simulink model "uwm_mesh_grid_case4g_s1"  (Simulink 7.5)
settings: Solver=ode45  StartTime=0.0  StopTime=8.0  RelTol=1e-4
undefined symbols (not defined in the file or in its folder): D1, Delta, dfilt, DiscIntNeverNeededParam
libraries: powerlib x90, powerlib_extras x24, dsparch4 x6
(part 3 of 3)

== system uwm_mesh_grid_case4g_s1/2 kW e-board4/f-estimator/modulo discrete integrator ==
  In1 : Inport
  Abs : Abs
  Constant1 : Constant  OutDataType=sfix(16)  OutScaling=2^0
  Discrete-Time Integrator : DiscreteIntegrator  ExternalReset=rising  InitialConditionSource=external  SampleTime=dt  OutDataType=fixdt(1, 16)  OutScaling=2^0  UpperSaturationLimit=100  LowerSaturationLimit=-100  ShowStatePort=on  ICPrevOutput=DiscIntNeverNeededParam  ICPrevScaledInput=DiscIntNeverNeededParam
  Gain1 : Gain  Gain=1+.0001  ParameterDataType=sfix(16)  ParameterScaling=2^0  OutDataType=sfix(16)  OutScaling=2^0
  IC : InitialCondition  Value=0
  Math Function : Math  Operator=rem  OutDataType=sfix(16)  OutScaling=2^0
  Relational Operator : RelationalOperator
  Out1 : Outport
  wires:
  Math Function/1 -> IC/1
  IC/1 -> Discrete-Time Integrator/3
  Discrete-Time Integrator/1 -> Out1/1
  In1/1 -> Discrete-Time Integrator/1
  Abs/1 -> Math Function/1, Relational Operator/1
  Constant1/1 -> Math Function/2, Relational Operator/2
  Gain1/1 -> Abs/1
  Discrete-Time Integrator/State -> Gain1/1
  Relational Operator/1 -> Discrete-Time Integrator/2

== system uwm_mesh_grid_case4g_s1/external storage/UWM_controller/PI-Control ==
  In1 : Inport
  Gain : Gain  Gain=.01  ParameterDataType=sfix(16)  ParameterScaling=2^0  OutDataType=sfix(16)  OutScaling=2^0
  Gain1 : Gain  Gain=5  ParameterDataType=sfix(16)  ParameterScaling=2^0  OutDataType=sfix(16)  OutScaling=2^0
  Gain2 : Gain  Gain=750  ParameterDataType=sfix(16)  ParameterScaling=2^0  OutDataType=sfix(16)  OutScaling=2^0
  Integrator1 : Integrator  LimitOutput=on  UpperSaturationLimit=1000  LowerSaturationLimit=-1000
  Sum4 : Sum  Inputs=|++  OutDataType=sfix(16)  OutScaling=2^0
  Out1 : Outport
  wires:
  Gain/1 -> Sum4/1
  Integrator1/1 -> Sum4/2
  In1/1 -> Gain1/1, Gain/1
  Gain1/1 -> Integrator1/1
  Sum4/1 -> Gain2/1
  Gain2/1 -> Out1/1

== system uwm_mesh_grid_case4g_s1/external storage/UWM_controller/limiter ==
  In1 : Inport
  Integrator1 : Integrator  LimitOutput=on  UpperSaturationLimit=0  LowerSaturationLimit=-pi
  Integrator2 : Integrator  LimitOutput=on  UpperSaturationLimit=pi  LowerSaturationLimit=0
  Kilim : Gain  Gain=30  ParameterDataType=sfix(16)  ParameterScaling=2^0  OutDataType=sfix(16)  OutScaling=2^0
  Kilim1 : Gain  Gain=30  ParameterDataType=sfix(16)  ParameterScaling=2^0  OutDataType=sfix(16)  OutScaling=2^0
  Kplim : Gain  Gain=3  ParameterDataType=sfix(16)  ParameterScaling=2^0  OutDataType=sfix(16)  OutScaling=2^0
  Kplim1 : Gain  Gain=3  ParameterDataType=sfix(16)  ParameterScaling=2^0  OutDataType=sfix(16)  OutScaling=2^0
  Plimit : Constant  Value=1.0  OutDataType=sfix(16)  OutScaling=2^0
  Plimit1 : Constant  Value=-.1667  OutDataType=sfix(16)  OutScaling=2^0
  Saturation1 : Saturate  UpperLimit=pi  LowerLimit=0  OutDataType=fixdt(1, 16)  OutScaling=2^0
  Saturation2 : Saturate  UpperLimit=0  LowerLimit=-pi  OutDataType=fixdt(1, 16)  OutScaling=2^0
  Sum1 : Sum  Inputs=-+|  OutDataType=sfix(16)  OutScaling=2^0
  Sum2 : Sum  Inputs=|++  OutDataType=sfix(16)  OutScaling=2^0
  Sum3 : Sum  OutDataType=sfix(16)  OutScaling=2^0
  Sum4 : Sum  Inputs=|+-  OutDataType=sfix(16)  OutScaling=2^0
  Sum9 : Sum  Inputs=|++  OutDataType=sfix(16)  OutScaling=2^0
  Out1 : Outport
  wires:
  Sum3/1 -> Out1/1
  Plimit1/1 -> Sum1/2
  Integrator2/1 -> Sum2/2
  Kilim1/1 -> Integrator2/1
  Sum1/1 -> Kilim1/1, Kplim1/1
  In1/1 -> Sum1/1, Sum4/2
  Integrator1/1 -> Sum9/2
  Kilim/1 -> Integrator1/1
  Sum4/1 -> Kilim/1, Kplim/1
  Plimit/1 -> Sum4/1
  Kplim/1 -> Saturation2/1
  Saturation2/1 -> Sum9/1
  Sum9/1 -> Sum3/1
  Kplim1/1 -> Saturation1/1
  Saturation1/1 -> Sum2/1
  Sum2/1 -> Sum3/2

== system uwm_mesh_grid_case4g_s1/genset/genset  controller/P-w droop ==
  note: P
  P_req : Inport
  P : Inport  Port=2
  Sum2 : Sum  Inputs=+-|  OutDataType=sfix(16)  OutScaling=2^0
  Sum3 : Sum  Inputs=+++  OutDataType=sfix(16)  OutScaling=2^0
  k : Gain  Gain=1/pi  ParameterDataType=sfix(16)  ParameterScaling=2^0  OutDataType=sfix(16)  OutScaling=2^0
  limiter : Subsystem
  mP droop : Gain  Gain=pi  ParameterDataType=sfix(16)  ParameterScaling=2^0  OutDataType=sfix(16)  OutScaling=2^0
  rad2pu : Gain  Gain=1/(2*pi*60)  ParameterDataType=sfix(16)  ParameterScaling=2^0  OutDataType=sfix(16)  OutScaling=2^0
  w0 : Constant  Value=60*2*pi  OutDataType=fixdt(1, 16)  OutScaling=2^0
  w : Outport
  Pmm : Outport  Port=2
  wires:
  P_req/1 -> Sum2/1
  mP droop/1 -> Sum3/2
  limiter/1(Out1) -> Sum3/1, k/1
  w0/1 -> Sum3/3
  Sum2/1 -> mP droop/1
  P/1 -> limiter/1(In1), Sum2/2
  Sum3/1 -> rad2pu/1
  rad2pu/1 -> w/1
  k/1 -> Pmm/1

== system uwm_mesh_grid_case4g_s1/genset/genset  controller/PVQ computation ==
  note: P
  note: Q
  Vabc : Inport  OutDataType=fixdt(1, 16)  OutScaling=2^0
  Iabc : Inport  Port=2  OutDataType=fixdt(1, 16)  OutScaling=2^0
  " pu convert P" : Gain  Gain=1/Sbase  ParameterDataType=sfix(16)  ParameterScaling=2^0  OutDataType=sfix(16)  OutScaling=2^0
  " pu convert S" : Gain  Gain=1/Sbase  ParameterDataType=sfix(16)  ParameterScaling=2^0  OutDataType=sfix(16)  OutScaling=2^0
  " pu convert V" : Gain  Gain=1/(Vbase/sqrt(3))  ParameterDataType=sfix(16)  ParameterScaling=2^0  OutDataType=sfix(16)  OutScaling=2^0
  3-phase  Instantaneous  Active & Reactive Power : powerlib_extras/Measurements/3-phase  Instantaneous  Active & Reactive Power  DialogController=POWERSYS.PowerSysDialog  SystemSampleTime=-1
  Demux : Demux  Outputs=2
  RMS : Fcn  Expr=sqrt(u(1)*u(1)+u(2)*u(2)+u(3)*u(3))/sqrt(3)
  Transfer Fcn1 : TransferFcn  Denominator=[.01 1]
  Transfer Fcn2 : TransferFcn  Denominator=[.01 1]
  Transfer Fcn3 : TransferFcn  Denominator=[.01 1]
  P_pu : Outport  OutDataType=fixdt(1, 16)  OutScaling=2^0
  Vt : Outport  Port=2  OutDataType=fixdt(1, 16)  OutScaling=2^0
  Q_pu : Outport  Port=3  OutDataType=fixdt(1, 16)  OutScaling=2^0
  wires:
  Iabc/1 -> 3-phase  Instantaneous  Active & Reactive Power/2
  RMS/1 -> " pu convert V"/1
  Demux/2 -> " pu convert P"/1
  Demux/1 -> " pu convert S"/1
  3-phase  Instantaneous  Active & Reactive Power/1 -> Demux/1
  Vabc/1 -> RMS/1, 3-phase  Instantaneous  Active & Reactive Power/1
  Transfer Fcn1/1 -> P_pu/1
  " pu convert S"/1 -> Transfer Fcn1/1
  Transfer Fcn2/1 -> Q_pu/1
  " pu convert P"/1 -> Transfer Fcn2/1
  Transfer Fcn3/1 -> Vt/1
  " pu convert V"/1 -> Transfer Fcn3/1

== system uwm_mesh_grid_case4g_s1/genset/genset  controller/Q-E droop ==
  note: Q
  v_meas : Inport
  Q : Inport  Port=2
  E_req : Inport  Port=3
  PI-Control : Subsystem
  Sum : Sum  Inputs=|-+  OutDataType=sfix(16)  OutScaling=2^0
  Sum1 : Sum  Inputs=|+-  OutDataType=sfix(16)  OutScaling=2^0
  "mQ droop " : Gain  Gain=0.05  ParameterDataType=sfix(16)  ParameterScaling=2^0  OutDataType=sfix(16)  OutScaling=2^0
  Vpk : Outport
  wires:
  Sum1/1 -> PI-Control/1(In1)
  Sum/1 -> Sum1/1
  "mQ droop "/1 -> Sum/1
  PI-Control/1(Out1) -> Vpk/1
  Q/1 -> "mQ droop "/1
  E_req/1 -> Sum/2
  v_meas/1 -> Sum1/2

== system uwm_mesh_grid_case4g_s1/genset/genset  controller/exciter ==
  wr : Inport  OutDataType=fixdt(1, 16)  OutScaling=2^0
  Ef_mcd_wr : Inport  Port=2  OutDataType=fixdt(1, 16)  OutScaling=2^0
  Product : Product  OutDataType=fixdt(1, 16)  OutScaling=2^0
  Saturation : Saturate  UpperLimit=10  LowerLimit=-10  OutDataType=fixdt(1, 16)  OutScaling=2^0
  Transfer Fcn : TransferFcn  Denominator=[.001 1]
  Ef : Outport  OutDataType=fixdt(1, 16)  OutScaling=2^0
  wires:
  wr/1 -> Product/2
  Ef_mcd_wr/1 -> Product/1
  Product/1 -> Saturation/1
  Saturation/1 -> Transfer Fcn/1
  Transfer Fcn/1 -> Ef/1

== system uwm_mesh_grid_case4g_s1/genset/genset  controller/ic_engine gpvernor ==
  wr : Inport  OutDataType=fixdt(1, 16)  OutScaling=2^0
  Pmeas : Inport  Port=2  OutDataType=fixdt(1, 16)  OutScaling=2^0
  w : Inport  Port=3  OutDataType=fixdt(1, 16)  OutScaling=2^0
  IC_engine : Subsystem
  governor : Subsystem
  Pmech : Outport  OutDataType=fixdt(1, 16)  OutScaling=2^0
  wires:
  governor/1(fuel_cmd) -> IC_engine/1(fuel_cmd)
  Pmeas/1 -> governor/1(Pmeas)
  IC_engine/1(Pmech) -> Pmech/1
  wr/1 -> governor/3(wr), IC_engine/2(wr)
  w/1 -> governor/2(w)

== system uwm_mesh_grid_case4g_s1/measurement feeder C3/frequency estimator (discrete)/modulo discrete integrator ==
  In1 : Inport
  Abs : Abs
  Constant1 : Constant  OutDataType=sfix(16)  OutScaling=2^0
  Discrete-Time Integrator : DiscreteIntegrator  ExternalReset=rising  InitialConditionSource=external  SampleTime=dt  OutDataType=fixdt(1, 16)  OutScaling=2^0  UpperSaturationLimit=100  LowerSaturationLimit=-100  ShowStatePort=on  ICPrevOutput=DiscIntNeverNeededParam  ICPrevScaledInput=DiscIntNeverNeededParam
  Gain1 : Gain  Gain=1+.0001  ParameterDataType=sfix(16)  ParameterScaling=2^0  OutDataType=sfix(16)  OutScaling=2^0
  IC : InitialCondition  Value=0
  Math Function : Math  Operator=rem  OutDataType=sfix(16)  OutScaling=2^0
  Relational Operator : RelationalOperator
  Out1 : Outport
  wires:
  Relational Operator/1 -> Discrete-Time Integrator/2
  Discrete-Time Integrator/State -> Gain1/1
  Gain1/1 -> Abs/1
  Constant1/1 -> Relational Operator/2, Math Function/2
  Abs/1 -> Relational Operator/1, Math Function/1
  In1/1 -> Discrete-Time Integrator/1
  Discrete-Time Integrator/1 -> Out1/1
  IC/1 -> Discrete-Time Integrator/3
  Math Function/1 -> IC/1

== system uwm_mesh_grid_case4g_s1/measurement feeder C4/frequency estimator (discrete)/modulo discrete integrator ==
  In1 : Inport
  Abs : Abs
  Constant1 : Constant  OutDataType=sfix(16)  OutScaling=2^0
  Discrete-Time Integrator : DiscreteIntegrator  ExternalReset=rising  InitialConditionSource=external  SampleTime=dt  OutDataType=fixdt(1, 16)  OutScaling=2^0  UpperSaturationLimit=100  LowerSaturationLimit=-100  ShowStatePort=on  ICPrevOutput=DiscIntNeverNeededParam  ICPrevScaledInput=DiscIntNeverNeededParam
  Gain1 : Gain  Gain=1+.0001  ParameterDataType=sfix(16)  ParameterScaling=2^0  OutDataType=sfix(16)  OutScaling=2^0
  IC : InitialCondition  Value=0
  Math Function : Math  Operator=rem  OutDataType=sfix(16)  OutScaling=2^0
  Relational Operator : RelationalOperator
  Out1 : Outport
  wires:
  Relational Operator/1 -> Discrete-Time Integrator/2
  Discrete-Time Integrator/State -> Gain1/1
  Gain1/1 -> Abs/1
  Constant1/1 -> Relational Operator/2, Math Function/2
  Abs/1 -> Relational Operator/1, Math Function/1
  In1/1 -> Discrete-Time Integrator/1
  Discrete-Time Integrator/1 -> Out1/1
  IC/1 -> Discrete-Time Integrator/3
  Math Function/1 -> IC/1

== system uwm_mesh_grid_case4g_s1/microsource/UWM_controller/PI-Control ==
  In1 : Inport
  Gain : Gain  Gain=.01  ParameterDataType=sfix(16)  ParameterScaling=2^0  OutDataType=sfix(16)  OutScaling=2^0
  Gain1 : Gain  Gain=5  ParameterDataType=sfix(16)  ParameterScaling=2^0  OutDataType=sfix(16)  OutScaling=2^0
  Gain2 : Gain  Gain=750  ParameterDataType=sfix(16)  ParameterScaling=2^0  OutDataType=sfix(16)  OutScaling=2^0
  Integrator1 : Integrator  LimitOutput=on  UpperSaturationLimit=100  LowerSaturationLimit=-100  ZeroCross=off
  Sum4 : Sum  Inputs=|++  OutDataType=sfix(16)  OutScaling=2^0
  Out1 : Outport
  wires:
  Gain/1 -> Sum4/1
  Integrator1/1 -> Sum4/2
  In1/1 -> Gain1/1, Gain/1
  Gain1/1 -> Integrator1/1
  Sum4/1 -> Gain2/1
  Gain2/1 -> Out1/1

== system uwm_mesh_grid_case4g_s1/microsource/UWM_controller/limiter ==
  In1 : Inport
  Integrator1 : Integrator  LimitOutput=on  UpperSaturationLimit=0  LowerSaturationLimit=-pi  ZeroCross=off
  Integrator2 : Integrator  LimitOutput=on  UpperSaturationLimit=pi  LowerSaturationLimit=0  ZeroCross=off
  Kilim : Gain  Gain=30  ParameterDataType=sfix(16)  ParameterScaling=2^0  OutDataType=sfix(16)  OutScaling=2^0
  Kilim1 : Gain  Gain=30  ParameterDataType=sfix(16)  ParameterScaling=2^0  OutDataType=sfix(16)  OutScaling=2^0
  Kplim : Gain  Gain=3  ParameterDataType=sfix(16)  ParameterScaling=2^0  OutDataType=sfix(16)  OutScaling=2^0
  Kplim1 : Gain  Gain=3  ParameterDataType=sfix(16)  ParameterScaling=2^0  OutDataType=sfix(16)  OutScaling=2^0
  Plimit : Constant  Value=1.0  OutDataType=sfix(16)  OutScaling=2^0
  Plimit1 : Constant  Value=0.0  OutDataType=sfix(16)  OutScaling=2^0
  Saturation1 : Saturate  UpperLimit=pi  LowerLimit=0  OutDataType=fixdt(1, 16)  OutScaling=2^0
  Saturation2 : Saturate  UpperLimit=0  LowerLimit=-pi  OutDataType=fixdt(1, 16)  OutScaling=2^0
  Sum1 : Sum  Inputs=-+|  OutDataType=sfix(16)  OutScaling=2^0
  Sum2 : Sum  Inputs=|++  OutDataType=sfix(16)  OutScaling=2^0
  Sum3 : Sum  OutDataType=sfix(16)  OutScaling=2^0
  Sum4 : Sum  Inputs=|+-  OutDataType=sfix(16)  OutScaling=2^0
  Sum9 : Sum  Inputs=|++  OutDataType=sfix(16)  OutScaling=2^0
  Out1 : Outport
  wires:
  Sum3/1 -> Out1/1
  Plimit1/1 -> Sum1/2
  Integrator2/1 -> Sum2/2
  Kilim1/1 -> Integrator2/1
  Sum1/1 -> Kilim1/1, Kplim1/1
  In1/1 -> Sum1/1, Sum4/2
  Integrator1/1 -> Sum9/2
  Kilim/1 -> Integrator1/1
  Sum4/1 -> Kilim/1, Kplim/1
  Plimit/1 -> Sum4/1
  Kplim1/1 -> Saturation1/1
  Saturation1/1 -> Sum2/1
  Kplim/1 -> Saturation2/1
  Saturation2/1 -> Sum9/1
  Sum9/1 -> Sum3/1
  Sum2/1 -> Sum3/2

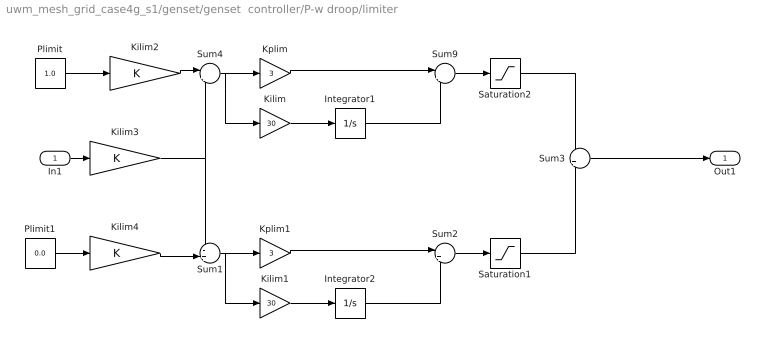
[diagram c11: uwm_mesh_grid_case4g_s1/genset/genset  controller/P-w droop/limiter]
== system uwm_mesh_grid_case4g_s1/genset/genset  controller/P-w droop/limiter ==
  In1 : Inport
  Integrator1 : Integrator  UpperSaturationLimit=0  LowerSaturationLimit=-2*pi
  Integrator2 : Integrator  UpperSaturationLimit=2*pi  LowerSaturationLimit=0
  Kilim : Gain  Gain=30  ParameterDataType=sfix(16)  ParameterScaling=2^0  OutDataType=sfix(16)  OutScaling=2^0
  Kilim1 : Gain  Gain=30  ParameterDataType=sfix(16)  ParameterScaling=2^0  OutDataType=sfix(16)  OutScaling=2^0
  Kilim2 : Gain  ParameterDataType=sfix(16)  ParameterScaling=2^0  OutDataType=sfix(16)  OutScaling=2^0
  Kilim3 : Gain  ParameterDataType=sfix(16)  ParameterScaling=2^0  OutDataType=sfix(16)  OutScaling=2^0
  Kilim4 : Gain  ParameterDataType=sfix(16)  ParameterScaling=2^0  OutDataType=sfix(16)  OutScaling=2^0
  Kplim : Gain  Gain=3  ParameterDataType=sfix(16)  ParameterScaling=2^0  OutDataType=sfix(16)  OutScaling=2^0
  Kplim1 : Gain  Gain=3  ParameterDataType=sfix(16)  ParameterScaling=2^0  OutDataType=sfix(16)  OutScaling=2^0
  Plimit : Constant  Value=1.0  OutDataType=sfix(16)  OutScaling=2^0
  Plimit1 : Constant  Value=0.0  OutDataType=sfix(16)  OutScaling=2^0
  Saturation1 : Saturate  UpperLimit=pi  LowerLimit=0  OutDataType=fixdt(1, 16)  OutScaling=2^0
  Saturation2 : Saturate  UpperLimit=0  LowerLimit=-pi  OutDataType=fixdt(1, 16)  OutScaling=2^0
  Sum1 : Sum  Inputs=-+|  OutDataType=sfix(16)  OutScaling=2^0
  Sum2 : Sum  Inputs=|++  OutDataType=sfix(16)  OutScaling=2^0
  Sum3 : Sum  OutDataType=sfix(16)  OutScaling=2^0
  Sum4 : Sum  Inputs=|+-  OutDataType=sfix(16)  OutScaling=2^0
  Sum9 : Sum  Inputs=|++  OutDataType=sfix(16)  OutScaling=2^0
  Out1 : Outport
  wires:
  Sum3/1 -> Out1/1
  Saturation2/1 -> Sum3/1
  Saturation1/1 -> Sum3/2
  Sum2/1 -> Saturation1/1
  Integrator2/1 -> Sum2/2
  Kplim1/1 -> Sum2/1
  Kilim1/1 -> Integrator2/1
  Sum1/1 -> Kilim1/1, Kplim1/1
  Sum9/1 -> Saturation2/1
  Integrator1/1 -> Sum9/2
  Kplim/1 -> Sum9/1
  Kilim/1 -> Integrator1/1
  Sum4/1 -> Kilim/1, Kplim/1
  Kilim2/1 -> Sum4/1
  Plimit/1 -> Kilim2/1
  In1/1 -> Kilim3/1
  Kilim3/1 -> Sum4/2, Sum1/1
  Plimit1/1 -> Kilim4/1
  Kilim4/1 -> Sum1/2

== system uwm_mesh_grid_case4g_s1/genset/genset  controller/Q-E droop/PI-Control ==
  In1 : Inport
  Constant1 : Constant  OutDataType=fixdt(1, 16)  OutScaling=2^0
  Gain : Gain  Gain=1000  ParameterDataType=sfix(16)  ParameterScaling=2^0  OutDataType=sfix(16)  OutScaling=2^0
  Gain1 : Gain  Gain=10  ParameterDataType=sfix(16)  ParameterScaling=2^0  OutDataType=sfix(16)  OutScaling=2^0
  Integrator1 : Integrator  InitialCondition=.88  UpperSaturationLimit=1  LowerSaturationLimit=-1
  Sum1 : Sum  Inputs=|++  OutDataType=sfix(16)  OutScaling=2^0
  Sum4 : Sum  Inputs=|++  OutDataType=sfix(16)  OutScaling=2^0
  Out1 : Outport
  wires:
  Gain/1 -> Sum4/1
  Integrator1/1 -> Sum4/2
  In1/1 -> Gain1/1, Gain/1
  Gain1/1 -> Integrator1/1
  Sum1/1 -> Out1/1
  Sum4/1 -> Sum1/1
  Constant1/1 -> Sum1/2

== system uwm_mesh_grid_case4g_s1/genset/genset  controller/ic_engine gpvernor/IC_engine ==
  fuel_cmd : Inport  OutDataType=fixdt(1, 16)  OutScaling=2^0
  wr : Inport  Port=2  OutDataType=fixdt(1, 16)  OutScaling=2^0
  Delay : TransportDelay  DelayTime=.022
  Friction_losses : Fcn  Expr=u(1)*u(1)*u(2)
  Fuel_torque : Fcn  Expr=u(1)*3.6*11.8238*0.47*1000
  Mux : Mux  Inputs=2
  Mux1 : Mux  Inputs=2
  Power Limit : Saturate  UpperLimit=1  LowerLimit=0  OutDataType=fixdt(1, 16)  OutScaling=2^0
  Sum : Sum  Inputs=|+-  OutDataType=fixdt(1, 16)  OutScaling=2^0
  Torque_to_power_pu : Fcn  Expr=u(1)*u(2)/12500
  mech_losses : Constant  Value=0.36  OutDataType=fixdt(1, 16)  OutScaling=2^0
  Pmech : Outport  OutDataType=fixdt(1, 16)  OutScaling=2^0
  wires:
  Fuel_torque/1 -> Delay/1
  fuel_cmd/1 -> Fuel_torque/1
  Delay/1 -> Mux/1
  wr/1 -> Mux/2, Mux1/1
  mech_losses/1 -> Mux1/2
  Mux1/1 -> Friction_losses/1
  Mux/1 -> Torque_to_power_pu/1
  Torque_to_power_pu/1 -> Sum/1
  Friction_losses/1 -> Sum/2
  Sum/1 -> Power Limit/1
  Power Limit/1 -> Pmech/1

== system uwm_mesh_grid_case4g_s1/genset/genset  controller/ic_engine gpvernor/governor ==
  Pmeas : Inport  OutDataType=fixdt(1, 16)  OutScaling=2^0
  w : Inport  Port=2  OutDataType=fixdt(1, 16)  OutScaling=2^0
  wr : Inport  Port=3  OutDataType=fixdt(1, 16)  OutScaling=2^0
  Gain : Gain  Gain=20  ParameterDataType=fixdt(1, 16)  ParameterScaling=2^0  OutDataType=fixdt(1, 16)  OutScaling=2^0
  Gain1 : Gain  Gain=10  ParameterDataType=fixdt(1, 16)  ParameterScaling=2^0  OutDataType=fixdt(1, 16)  OutScaling=2^0
  Integrator : Integrator  LimitOutput=on  UpperSaturationLimit=10  LowerSaturationLimit=-10
  Sum : Sum  Inputs=-+|  OutDataType=fixdt(1, 16)  OutScaling=2^0
  Sum1 : Sum  Inputs=++|  OutDataType=fixdt(1, 16)  OutScaling=2^0
  Sum2 : Sum  Inputs=++|  OutDataType=fixdt(1, 16)  OutScaling=2^0
  Te_cmd_t0_fuel : Fcn  Expr=u(1)/1.6
  Torque_limit : Saturate  UpperLimit=1000  LowerLimit=-1000  OutDataType=fixdt(1, 16)  OutScaling=2^0
  fuel_cmd : Outport  OutDataType=fixdt(1, 16)  OutScaling=2^0
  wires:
  w/1 -> Sum/2
  wr/1 -> Sum/1
  Sum/1 -> Integrator/1, Gain1/1
  Integrator/1 -> Gain/1
  Gain/1 -> Sum1/1
  Gain1/1 -> Sum1/2
  Pmeas/1 -> Sum2/1
  Sum1/1 -> Sum2/2
  Sum2/1 -> Torque_limit/1
  Torque_limit/1 -> Te_cmd_t0_fuel/1
  Te_cmd_t0_fuel/1 -> fuel_cmd/1
